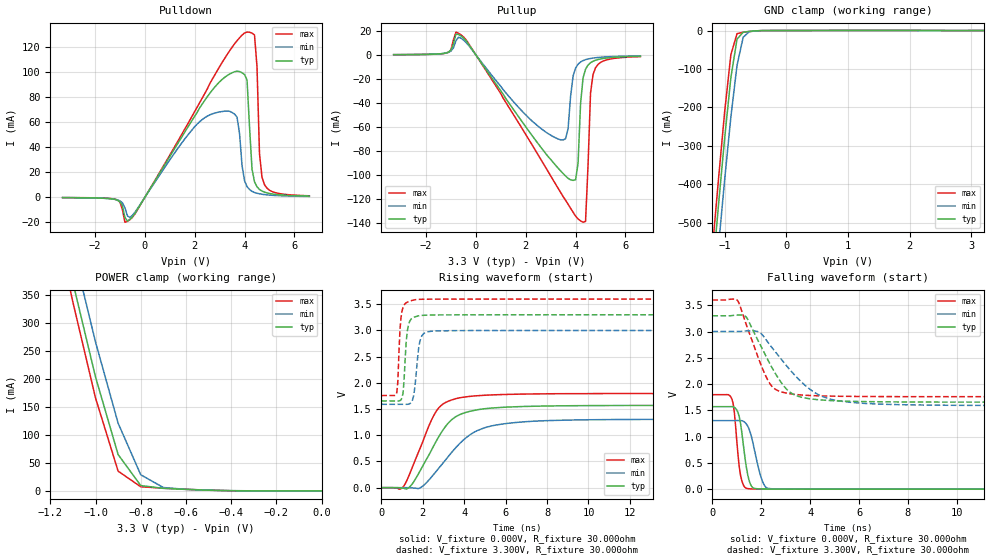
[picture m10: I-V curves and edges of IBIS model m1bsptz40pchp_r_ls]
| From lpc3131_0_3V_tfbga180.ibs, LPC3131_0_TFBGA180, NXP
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| |   Rev 0.20 IBIS Model Design Automation Generation   |
| |   N O N - S I L I C O N   C O R R E L A T E D   |
| |   This IBIS [Model] is pre-Beta tactical support   |
| |  Note: this IBIS [Model] contains clamp curves generated   |
| |   through simulation which should not be relied upon   |
| Date/Time   : 2010 Jan 25 (Mon) 11:58:19
| Pccmos090 jliolib_p50 2.0
|   0.9 um 3.3V pad library
|   seven level metal
|   dual oxide
|   dual threshold voltage
|   nominal line mixed supply
|   parasitic extracted netlists
| Process block a10
| mem1bsptz40pchp
|   Bidirectional Pad 3.3
|   3state Output
|   Plain Input
|   CMOS
|   Programmable between
|   - (p1=0, p2=1) plain input
|   - (p1=0, p2=0) with Pull Up
|   - (p1=1, p2=1) with Pull Down
|   - (p1=1, p2=0) with Repeater
| Repeater Mode low power(esh=1, p1=1, p2=0)
[Model]   m1bsptz40pchp_r_ls | of mem1bsptz40pchp
Model_type   I/O
Polarity   Non-Inverting
Enable   Active-Low
|  Reciever Thresholds
Vinl   = 0.99V
Vinh   = 2.31V
| AC Test Load Conditions
Vref   = 0
Cref   = 0
Rref   = 1000000000
Vmeas   = 1.65
| [Process Range]   typical   min   max
| C_comp edge width   400.000ps   400.000ps   400.000ps
| C_comp Tstrobe   40.000fs   40.000fs   40.000fs
C_comp   200.000pF   200.000pF   200.000pF
[Temperature Range]   25   125   -40
[Voltage Range]   3.30V   3.00V   3.60V
[GND Clamp Reference]   0.00V   0.00V   0.00V
[Pulldown Reference]   0.00V   0.00V   0.00V
[POWER Clamp Reference]   3.30V   3.00V   3.60V
[Pullup Reference]   3.30V   3.00V   3.60V
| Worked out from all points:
|   slope of the pulldown table from 0 to 0.495 V, typ, clamps not added: 30.9 ohm
|   slope of the pullup table from 0 to 0.495 V, typ, clamps not added: 33.4 ohm
|   GND clamp passes 1 mA (typ) near -0.51 V on its own axis
|   POWER clamp passes 1 mA (typ) near -0.47 V on its own axis
|   rising waveform, V_fixture 0.000V, R_fixture 30.000ohm: 20-80 % time 1.43ns typ, 1.87ns min, 1.15ns max; typ from 0 V to 1.57 V
|   falling waveform, V_fixture 0.000V, R_fixture 30.000ohm: 20-80 % time 280ps typ, 398ps min, 217ps max; typ from 1.57 V to 0 V
|   rising waveform, V_fixture 3.300V, R_fixture 30.000ohm: 20-80 % time 165ps typ, 222ps min, 139ps max; typ from 1.66 V to 3.3 V
|   falling waveform, V_fixture 3.300V, R_fixture 30.000ohm: 20-80 % time 1.17ns typ, 1.68ns min, 898ps max; typ from 3.3 V to 1.66 V
[GND Clamp]
| ref voltage   0.00V   0.00V   0.00V
|   Voltage   I(typ)   I(min)   I(max)
-3.3V     -4.732A    -4.814A    -4.684A
-1.2V     -636mA     -742.5mA   -569.7mA
-1.1V     -453.5mA   -561.8mA   -385.7mA
-1V       -279mA     -387.5mA   -210.8mA
-900mV    -122.8mA   -225.5mA   -63.13mA
-800mV    -22.45mA   -90.49mA   -8.204mA
-700mV    -4.394mA   -17.31mA   -4.534mA
-600mV    -2.163mA   -3.055mA   -2.529mA
-300mV    -78.17uA   -69.01uA   -98.11uA
3.2V      -17.82uA   34.39uA    -87.56uA
[Power Clamp]   | Vtable = Vcc - Vpad
| ref voltage   3.30V   3.00V   3.60V
|   Voltage   I(typ)   I(min)   I(max)
-3.3V     4.647A     4.675A     4.636A
-1.2V     553.3mA    610.4mA    520.8mA
-1.1V     373.2mA    433.6mA    337.9mA
-1V       204mA      266.6mA    166.4mA
-900mV    65.07mA    121.2mA    35.4mA
-800mV    9.632mA    28.93mA    7.456mA
-700mV    4.576mA    6.079mA    4.901mA
-600mV    2.711mA    2.826mA    2.897mA
-400mV    366.5uA    549.1uA    304.5uA
0V        388.1pA    9.875nA    264.4pA
[Pulldown]
| ref voltage   0.00V   0.00V   0.00V
|   Voltage   I(typ)   I(min)   I(max)
-3.3V     -236.7uA   -252.6uA   -192uA
-1.2V     -1.652mA   -1.556mA   -1.496mA
-600mV    -17.54mA   -16.01mA   -17.75mA
2.9V      89.88mA    67.56mA    100.6mA
3.7V      100.4mA    63.73mA    124.7mA
4.1V      93.46mA    8.514mA    131.5mA
4.3V      22.53mA    4.741mA    130.7mA
4.4V      12.45mA    3.859mA    129.3mA
4.5V      8.406mA    3.243mA    104mA
4.6V      6.249mA    2.791mA    34.96mA
4.8V      4.128mA    2.175mA    10.1mA
6.6V      975.1uA    710uA      1.222mA
[Pullup]   | Vtable = Vcc - Vpad
| ref voltage   3.30V   3.00V   3.60V
|   Voltage   I(typ)   I(min)   I(max)
-3.3V     206.8uA    209.1uA    174.1uA
-500mV    14.05mA    12.42mA    15mA
3.4V      -96.32mA   -70.52mA   -114.2mA
3.7V      -102.5mA   -61.11mA   -124.1mA
3.9V      -104.2mA   -17.59mA   -130.7mA
4.1V      -89.97mA   -7.665mA   -136.3mA
4.2V      -40.47mA   -5.865mA   -137.9mA
4.3V      -19.14mA   -4.724mA   -138.9mA
4.4V      -11.89mA   -3.942mA   -138.3mA
4.6V      -6.502mA   -2.948mA   -31.69mA
4.7V      -5.28mA    -2.614mA   -16.33mA
6.6V      -1.118mA   -810uA     -1.413mA
[Ramp]
R_load   = 30.000ohm
|   dV/dt(typ)   dV/dt(min)   dV/dt(max)
dV/dt_r   941.954mV/1.400ns   783.272mV/1.900ns   1.079V/1.150ns
dV/dt_f   986.681mV/1.150ns   845.135mV/1.700ns   1.104V/900.000ps
[Rising Waveform]  | cubic spline decimation from 501 points
V_fixture   = 0.000V
R_fixture   = 30.000ohm
|   Time   V(typ)   V(min)   V(max)
0s        3.993nV    181.6nV    2.818nV
950ps     -5.394mV   33.03uV    -20.12mV
1.35ns    8.653mV    -1.865mV   245.1mV
1.9ns     341.7mV    2.846mV    778.9mV
2.65ns    887.5mV    312mV      1.458V
3.2ns     1.218V     578.3mV    1.644V
3.8ns     1.397V     849.1mV    1.717V
5.05ns    1.509V     1.151V     1.765V
7.35ns    1.554V     1.269V     1.789V
25ns      1.57V      1.305V     1.798V
[Falling Waveform]  | cubic spline decimation from 501 points
V_fixture   = 0.000V
R_fixture   = 30.000ohm
|   Time   V(typ)   V(min)   V(max)
0s        1.57V      1.305V     1.798V
800ps     1.571V     1.305V     1.715V
900ps     1.557V     1.305V     1.459V
1.05ns    1.456V     1.306V     646.7mV
1.15ns    1.258V     1.306V     268.5mV
1.45ns    265.2mV    1.196V     10.51mV
1.65ns    29.88mV    899.7mV    4.358mV
2ns       4.319mV    214.4mV    2.011mV
2.35ns    2.284mV    10.47mV    802.6uV
25ns      18.42nV    233nV      24.45nV
[Rising Waveform]  | cubic spline decimation from 501 points
V_fixture   = 3.300V
V_fixture_min = 3.000V
V_fixture_max = 3.600V
R_fixture   = 30.000ohm
|   Time   V(typ)   V(min)   V(max)
0s        1.656V     1.591V     1.759V
750ps     1.655V     1.591V     1.818V
900ps     1.662V     1.591V     3.011V
1ns       1.712V     1.591V     3.372V
1.25ns    2.977V     1.591V     3.54V
1.5ns     3.239V     1.668V     3.576V
1.65ns    3.263V     2.038V     3.589V
1.9ns     3.286V     2.847V     3.596V
2.4ns     3.296V     2.985V     3.598V
25ns      3.3V       3V         3.6V
[Falling Waveform]  | cubic spline decimation from 501 points
V_fixture   = 3.300V
V_fixture_min = 3.000V
V_fixture_max = 3.600V
R_fixture   = 30.000ohm
|   Time   V(typ)   V(min)   V(max)
0s        3.3V       3V         3.6V
1ns       3.313V     3V         3.604V
1.35ns    3.291V     3.01V      3.183V
1.95ns    2.754V     2.976V     2.412V
2.35ns    2.389V     2.747V     2.011V
2.65ns    2.146V     2.571V     1.883V
3.2ns     1.837V     2.258V     1.814V
4.45ns    1.698V     1.773V     1.775V
6.2ns     1.667V     1.633V     1.764V
25ns      1.656V     1.591V     1.759V
